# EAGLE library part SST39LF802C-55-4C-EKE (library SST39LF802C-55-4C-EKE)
FLASH Memory IC 8Mbit Parallel 55 ns 48-TSOP 3V ~ 3.6V,55 ns,10s 0C ~ 70C (TA) Source: Datasheet
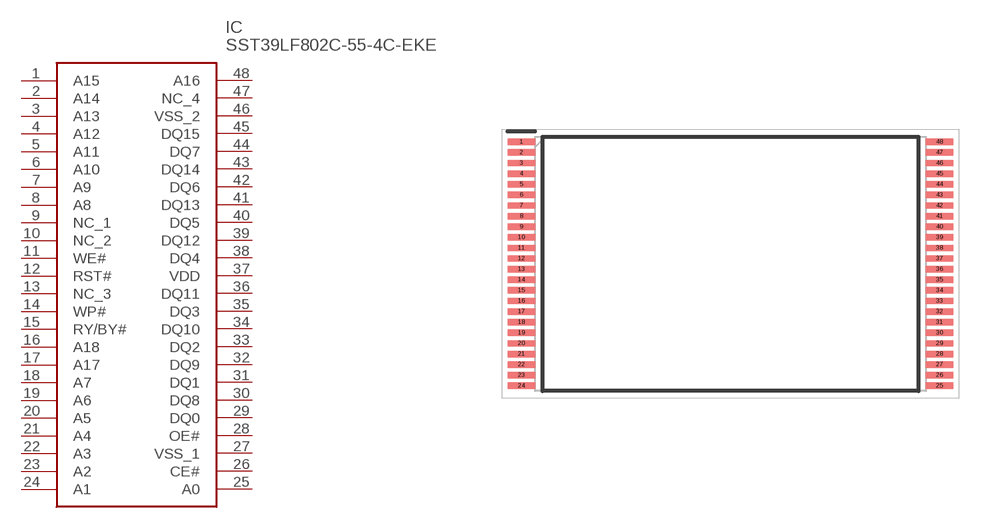
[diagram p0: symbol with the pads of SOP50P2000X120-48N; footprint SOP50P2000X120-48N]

Designator prefix IC

## SST39LF802C-55-4C-EKE (Description: FLASH Memory IC 8Mbit Parallel 55 ns 48-TSOP 3V ~ 3.6V,55 ns,10s 0C ~ 70C (TA); Height: 1.2mm; Manufacturer_Name: Microchip; Manufacturer_Part_Number: SST39LF802C-55-4C-EKE; Mouser_Part_Number: 579-S39LF802C554CEKE; Mouser_Price-Stock: https://www.mouser.com/Search/Refine.aspx?Keyword=579-S39LF802C554CEKE)  [SOP50P2000X120-48N]
1  A15
2  A14
3  A13
4  A12
5  A11
6  A10
7  A9
8  A8
9  NC_1
10  NC_2
11  WE#
12  RST#
13  NC_3
14  WP#
15  RY/BY#
16  A18
17  A17
18  A7
19  A6
20  A5
21  A4
22  A3
23  A2
24  A1
25  A0
26  CE#
27  VSS_1
28  OE#
29  DQ0
30  DQ8
31  DQ1
32  DQ9
33  DQ2
34  DQ10
35  DQ3
36  DQ11
37  VDD
38  DQ4
39  DQ12
40  DQ5
41  DQ13
42  DQ6
43  DQ14
44  DQ7
45  DQ15
46  VSS_2
47  NC_4
48  A16

## Footprint SOP50P2000X120-48N (pad centres in mm)
48-lead Thin Small Outline Package (TSOP) 12mm x 20mm SST Package Code: EK
smd 1.3 x 0.3: 1 -9.85,5.75; 2 -9.85,5.25; 3 -9.85,4.75; 4 -9.85,4.25; 5 -9.85,3.75; 6 -9.85,3.25; 7 -9.85,2.75; 8 -9.85,2.25; 9 -9.85,1.75; 10 -9.85,1.25; 11 -9.85,0.75; 12 -9.85,0.25; 13 -9.85,-0.25; 14 -9.85,-0.75; 15 -9.85,-1.25; 16 -9.85,-1.75; 17 -9.85,-2.25; 18 -9.85,-2.75; 19 -9.85,-3.25; 20 -9.85,-3.75; 21 -9.85,-4.25; 22 -9.85,-4.75; 23 -9.85,-5.25; 24 -9.85,-5.75; 25 9.85,-5.75; 26 9.85,-5.25; 27 9.85,-4.75; 28 9.85,-4.25; 29 9.85,-3.75; 30 9.85,-3.25; 31 9.85,-2.75; 32 9.85,-2.25; 33 9.85,-1.75; 34 9.85,-1.25; 35 9.85,-0.75; 36 9.85,-0.25; 37 9.85,0.25; 38 9.85,0.75; 39 9.85,1.25; 40 9.85,1.75; 41 9.85,2.25; 42 9.85,2.75; 43 9.85,3.25; 44 9.85,3.75; 45 9.85,4.25; 46 9.85,4.75; 47 9.85,5.25; 48 9.85,5.75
